(* Logix 5000 AddOnInstructionDefinition export Banner_S15C_MEZ_PD_v2; software revision 32.00 *)

TYPE Banner_S15C_MEZ_Data_Set_0 :
STRUCT
   c1_c16 : INT;   // Channels 1 to 16
   c17_c32 : INT;   // Channels 17 to 32
   c33_c48 : INT;   // Channels 33 to 48
   c49_c64 : INT;   // Channels 49 to 64
   c65_c80 : INT;   // Channels 65 to 80
   c81_c96 : INT;   // Channels 81 to 96
   c97_c112 : INT;   // Channels 97 to 112
   c113_c128 : INT;   // Channels 113 to 128
   c129_c144 : INT;   // Channels 129 to 144
   c145_c160 : INT;   // Channels 145 to 160
   c161_c176 : INT;   // Channels 161 to 176
   c177_c192 : INT;   // Channels 177 to 192
   c193_c208 : INT;   // Channels 193 to 208
   c209_c224 : INT;   // Channels 209 to 224
   c225_c240 : INT;   // Channels 225 to 240
END_STRUCT
END_TYPE

TYPE Banner_S15C_MEZ_Data_Set_1 :
STRUCT
   FBB : DINT;   // First Beam Blocked
   LBB : DINT;   // Last Beam Blocked
   TBB : DINT;   // Total Beams Blocked
   TRN : DINT;   // Beam Transitions
   CBB : DINT;   // Contiguous Beams Blocked
   FBM : DINT;   // First Beam Made
   LBM : DINT;   // Last Beam Made
   TBM : DINT;   // Total Beams Made
   CBM : DINT;   // Contiguous Beams Made
   MBB : DINT;   // Middle Beam Blocked
   Emitter_Power : INT;
   Gain_Method : INT;
   Low_Sensitivity : INT;
   HW_Flag : INT;
   Number_of_Dirty_Channels : INT;
   Time_of_Servie : DINT;
END_STRUCT
END_TYPE

TYPE Banner_S15C_MEZ_Data_Set_2 :
STRUCT
   c241_c256 : INT;   // Channels 241 to 256
   c257_c272 : INT;   // Channels 257 to 272
   c273_c288 : INT;   // Channels 273 to 288
   c289_c304 : INT;   // Channels 289 to 304
   c305_c320 : INT;   // Channels 305 to 320
   c321_c336 : INT;   // Channels 321 to 336
   c337_c352 : INT;   // Channels 337 to 352
   c353_c368 : INT;   // Channels 353 to 368
   c369_c384 : INT;   // Channels 369 to 384
   c385_c400 : INT;   // Channels 385 to 400
   c401_c416 : INT;   // Channels 401 to 416
   c417_c432 : INT;   // Channels 417 to 432
   c433_c448 : INT;   // Channels 433 to 448
   c449_c464 : INT;   // Channels 448 to 464
   c465_c480 : INT;   // Channels 465 to 480
END_STRUCT
END_TYPE

TYPE Banner_S15C_MEZ_PDIO_v2 :   // UDT with all of the variables needed to control an IO-Link S15C MEZ.
STRUCT
   Read_Data_Set : SINT;   // 0 = VT English units, 1 = Metric units, 2 = Sensor Information
   Read_Status : SINT;   // 0 = failed, 1 = success
   Counter_Value : INT;
   Data_Set_0 : Banner_S15C_MEZ_Data_Set_0;   // English Data Set
   Data_Set_1 : Banner_S15C_MEZ_Data_Set_1;   // Metric Data Set
   Data_Set_2 : Banner_S15C_MEZ_Data_Set_2;   // Sensor Information Data Set
   DTI : SINT[32];   // Array with Raw Process data being transferred into AOI.
   Write_Data_Set : SINT;   // Set which Data Set should be gathered via the S15C.
END_STRUCT
END_TYPE

ADD_ON_INSTRUCTION Banner_S15C_MEZ_PD_v2   (* revision 2.0, vendor Banner Engineering *)
// AOI that used with the S15C MEZ sensor.
VAR_IN_OUT
   Process_Data : Banner_S15C_MEZ_PDIO_v2; {required}
END_VAR
VAR_INPUT
   Byte_Swap : BOOL; {required}
END_VAR
VAR
   Temp : INT[16]; {access None}
   W_Index : SINT; {access None}
   DT_Index : SINT; {access None}
   Data_Update : BOOL; {access None}
END_VAR

ROUTINE Logic   (* ladder *)
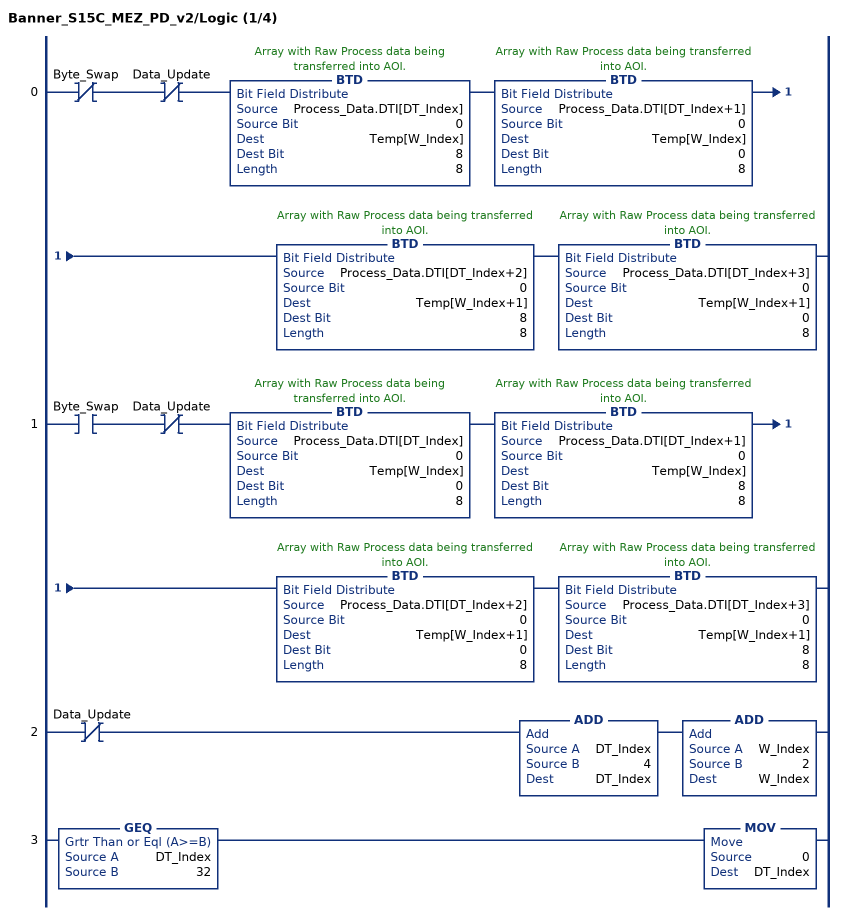
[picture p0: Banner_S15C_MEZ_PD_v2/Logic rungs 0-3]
   0: XIO(Byte_Swap)XIO(Data_Update)BTD(Process_Data.DTI[DT_Index],0,Temp[W_Index],8,8)BTD(Process_Data.DTI[DT_Index+1],0,Temp[W_Index],0,8)BTD(Process_Data.DTI[DT_Index+2],0,Temp[W_Index+1],8,8)BTD(Process_Data.DTI[DT_Index+3],0,Temp[W_Index+1],0,8);
   1: XIC(Byte_Swap)XIO(Data_Update)BTD(Process_Data.DTI[DT_Index],0,Temp[W_Index],0,8)BTD(Process_Data.DTI[DT_Index+1],0,Temp[W_Index],8,8)BTD(Process_Data.DTI[DT_Index+2],0,Temp[W_Index+1],0,8)BTD(Process_Data.DTI[DT_Index+3],0,Temp[W_Index+1],8,8);
   2: XIO(Data_Update)ADD(DT_Index,4,DT_Index)ADD(W_Index,2,W_Index);
   3: GEQ(DT_Index,32)MOV(0,DT_Index);
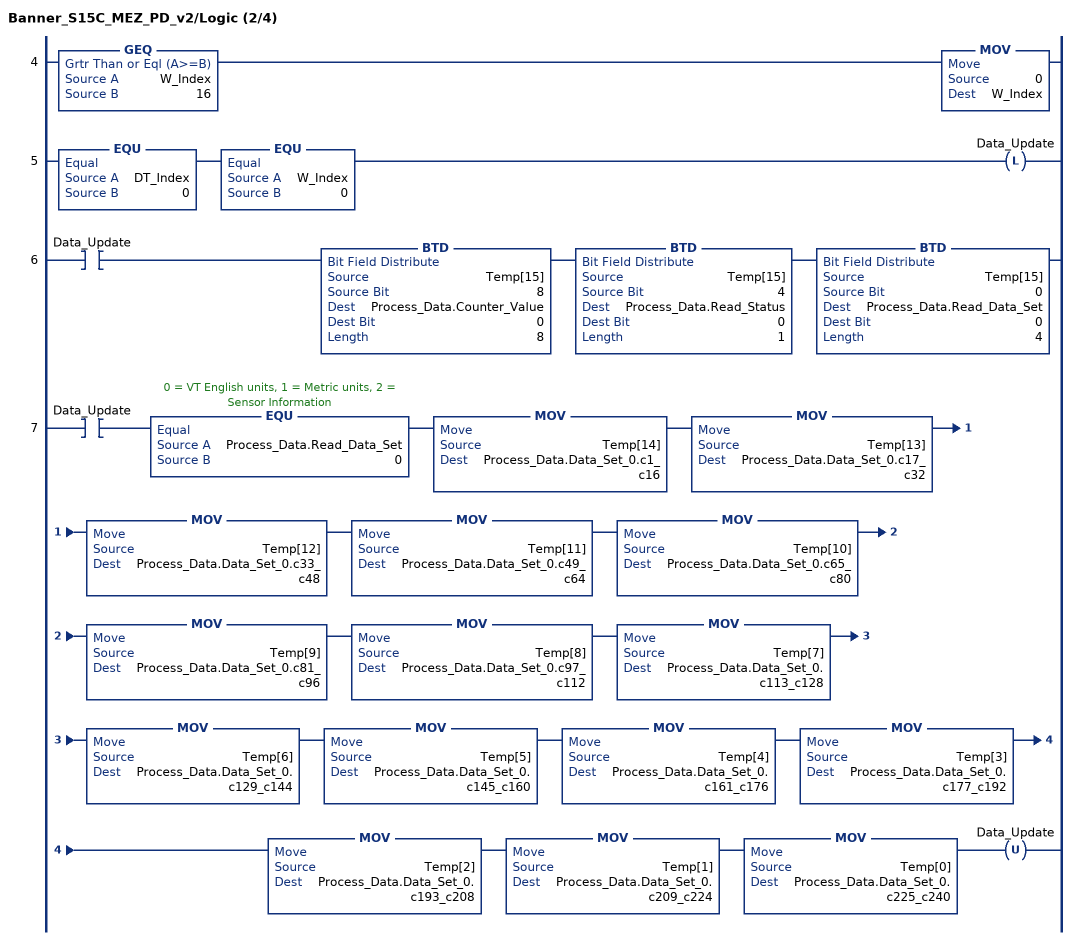
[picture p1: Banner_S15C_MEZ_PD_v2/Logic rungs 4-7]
   4: GEQ(W_Index,16)MOV(0,W_Index);
   5: EQU(DT_Index,0)EQU(W_Index,0)OTL(Data_Update);
   6: XIC(Data_Update)BTD(Temp[15],8,Process_Data.Counter_Value,0,8)BTD(Temp[15],4,Process_Data.Read_Status,0,1)BTD(Temp[15],0,Process_Data.Read_Data_Set,0,4);
   7: XIC(Data_Update)EQU(Process_Data.Read_Data_Set,0)MOV(Temp[14],Process_Data.Data_Set_0.c1_c16)MOV(Temp[13],Process_Data.Data_Set_0.c17_c32)MOV(Temp[12],Process_Data.Data_Set_0.c33_c48)MOV(Temp[11],Process_Data.Data_Set_0.c49_c64)MOV(Temp[10],Process_Data.Data_Set_0.c65_c80)MOV(Temp[9],Process_Data.Data_Set_0.c81_c96)MOV(Temp[8],Process_Data.Data_Set_0.c97_c112)MOV(Temp[7],Process_Data.Data_Set_0.c113_c128)MOV(Temp[6],Process_Data.Data_Set_0.c129_c144)MOV(Temp[5],Process_Data.Data_Set_0.c145_c160)MOV(Temp[4],Process_Data.Data_Set_0.c161_c176)MOV(Temp[3],Process_Data.Data_Set_0.c177_c192)MOV(Temp[2],Process_Data.Data_Set_0.c193_c208)MOV(Temp[1],Process_Data.Data_Set_0.c209_c224)MOV(Temp[0],Process_Data.Data_Set_0.c225_c240)OTU(Data_Update);
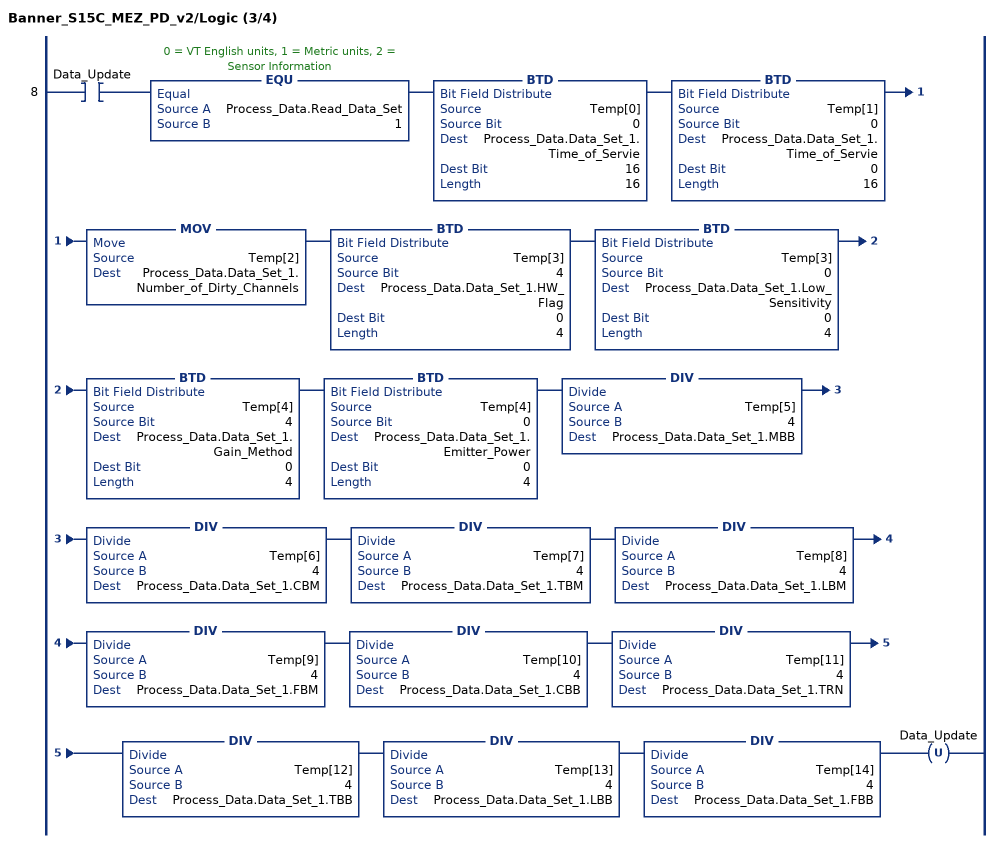
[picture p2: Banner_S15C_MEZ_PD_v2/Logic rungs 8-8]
   8: XIC(Data_Update)EQU(Process_Data.Read_Data_Set,1)BTD(Temp[0],0,Process_Data.Data_Set_1.Time_of_Servie,16,16)BTD(Temp[1],0,Process_Data.Data_Set_1.Time_of_Servie,0,16)MOV(Temp[2],Process_Data.Data_Set_1.Number_of_Dirty_Channels)BTD(Temp[3],4,Process_Data.Data_Set_1.HW_Flag,0,4)BTD(Temp[3],0,Process_Data.Data_Set_1.Low_Sensitivity,0,4)BTD(Temp[4],4,Process_Data.Data_Set_1.Gain_Method,0,4)BTD(Temp[4],0,Process_Data.Data_Set_1.Emitter_Power,0,4)DIV(Temp[5],4,Process_Data.Data_Set_1.MBB)DIV(Temp[6],4,Process_Data.Data_Set_1.CBM)DIV(Temp[7],4,Process_Data.Data_Set_1.TBM)DIV(Temp[8],4,Process_Data.Data_Set_1.LBM)DIV(Temp[9],4,Process_Data.Data_Set_1.FBM)DIV(Temp[10],4,Process_Data.Data_Set_1.CBB)DIV(Temp[11],4,Process_Data.Data_Set_1.TRN)DIV(Temp[12],4,Process_Data.Data_Set_1.TBB)DIV(Temp[13],4,Process_Data.Data_Set_1.LBB)DIV(Temp[14],4,Process_Data.Data_Set_1.FBB)OTU(Data_Update);
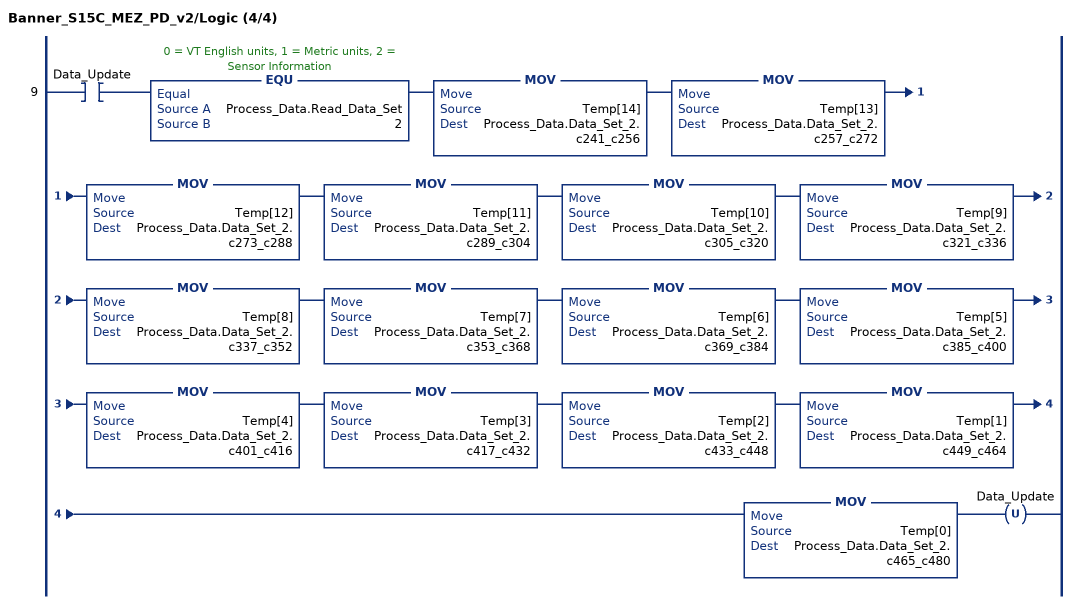
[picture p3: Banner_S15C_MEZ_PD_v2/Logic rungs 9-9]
   9: XIC(Data_Update)EQU(Process_Data.Read_Data_Set,2)MOV(Temp[14],Process_Data.Data_Set_2.c241_c256)MOV(Temp[13],Process_Data.Data_Set_2.c257_c272)MOV(Temp[12],Process_Data.Data_Set_2.c273_c288)MOV(Temp[11],Process_Data.Data_Set_2.c289_c304)MOV(Temp[10],Process_Data.Data_Set_2.c305_c320)MOV(Temp[9],Process_Data.Data_Set_2.c321_c336)MOV(Temp[8],Process_Data.Data_Set_2.c337_c352)MOV(Temp[7],Process_Data.Data_Set_2.c353_c368)MOV(Temp[6],Process_Data.Data_Set_2.c369_c384)MOV(Temp[5],Process_Data.Data_Set_2.c385_c400)MOV(Temp[4],Process_Data.Data_Set_2.c401_c416)MOV(Temp[3],Process_Data.Data_Set_2.c417_c432)MOV(Temp[2],Process_Data.Data_Set_2.c433_c448)MOV(Temp[1],Process_Data.Data_Set_2.c449_c464)MOV(Temp[0],Process_Data.Data_Set_2.c465_c480)OTU(Data_Update);
END_ROUTINE
END_ADD_ON_INSTRUCTION
